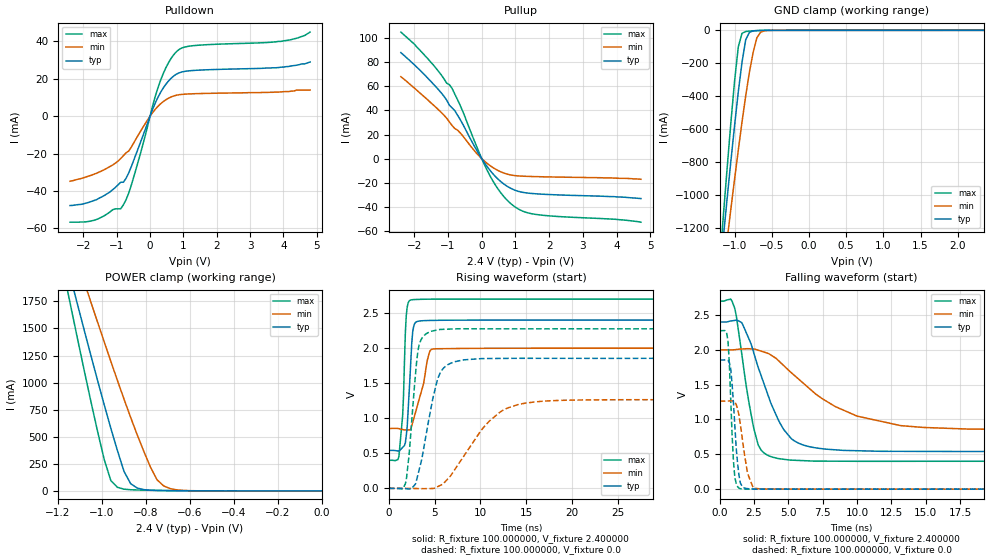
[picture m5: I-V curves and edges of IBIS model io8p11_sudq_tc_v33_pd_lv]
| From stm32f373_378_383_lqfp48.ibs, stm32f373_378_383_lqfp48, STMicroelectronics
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|   Model io8p11_sudq_tc_v33_pd_lv
[Model]  io8p11_sudq_tc_v33_pd_lv
Model_type I/O
Polarity   Non-Inverting
Enable   Active-Low
Vinl =   0.720000V
Vinh =   1.680000V
Vmeas =  1.200000V
Cref =   50.000000pF
Rref =   100.000000M
Vref =   0.0V
C_comp   1.373400pF   1.288200pF   1.481900pF
[Temperature Range]   25.000000   0.125000k   -40.000000
[Pullup Reference]   2.400000V   2.000000V   2.700000V
[Pulldown Reference]   0.0V   0.0V   0.0V
[POWER Clamp Reference]   2.400000V   2.000000V   2.700000V
[GND Clamp Reference]   0.0V   0.0V   0.0V
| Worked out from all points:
|   slope of the pulldown table from 0 to 0.36 V, typ, clamps not added: 25.7 ohm
|   slope of the pullup table from 0 to 0.36 V, typ, clamps not added: 26.8 ohm
|   GND clamp passes 1 mA (typ) near -0.67 V on its own axis
|   POWER clamp passes 1 mA (typ) near -0.60 V on its own axis
|   rising waveform, R_fixture 100.000000, V_fixture 2.400000: 20-80 % time 466ps typ, 1.22ns min, 428ps max; typ from 0.541 V to 2.4 V
|   rising waveform, R_fixture 100.000000, V_fixture 0.0: 20-80 % time 1.66ns typ, 4.33ns min, 861ps max; typ from 0 V to 1.85 V
|   falling waveform, R_fixture 100.000000, V_fixture 2.400000: 20-80 % time 2.12ns typ, 4.93ns min, 1.11ns max; typ from 2.4 V to 0.541 V
|   falling waveform, R_fixture 100.000000, V_fixture 0.0: 20-80 % time 392ps typ, 571ps min, 290ps max; typ from 1.85 V to 0 V
[Pulldown]
|Voltage   I(typ)   I(min)   I(max)
-2.4V     -47.8mA    -34.8mA    -56.7mA
-1.68V    -45.1mA    -31mA      -55.7mA
-1.12V    -39.3mA    -26.1mA    -50.03mA
-800mV    -35.33mA   -21.13mA   -47.42mA
-640mV    -30.33mA   -18.65mA   -41.16mA
-480mV    -23.12mA   -14mA      -31.94mA
240mV     10.22mA    5.339mA    15.38mA
480mV     17.22mA    8.864mA    26.1mA
800mV     22.59mA    11.27mA    34.68mA
1.36V     24.54mA    12.05mA    37.84mA
3.92V     26.2mA     13mA       40mA
4.8V      29mA       14mA       45mA
[Pullup]
|Voltage   I(typ)   I(min)   I(max)
-2.4V     88mA       68mA       105mA
-2V       77.9mA     58.6mA     95mA
-1.36V    59.6mA     42.6mA     75.1mA
-880mV    42.13mA    27.44mA    58.22mA
-560mV    28.45mA    18.75mA    39mA
-160mV    7.44mA     4.66mA     10.64mA
160mV     -6.607mA   -3.947mA   -9.704mA
480mV     -16.91mA   -9.806mA   -25.1mA
880mV     -24.89mA   -13.63mA   -37.75mA
1.2V      -27.87mA   -14.5mA    -43.37mA
1.6V      -29.13mA   -14.89mA   -46.24mA
4.72V     -33.1mA    -17.1mA    -52.7mA
[GND_clamp]
|Voltage   I(typ)   I(min)   I(max)
-2.4V     -7.358A    -6.372A    -8.78A
-1.2V     -1.489A    -1.65A     -1.416A
-1.15V    -1.254A    -1.461A    -1.124A
-1.1V     -1.024A    -1.273A    -838.2mA
-1.05V    -797.6mA   -1.088A    -563.2mA
-950mV    -374.6mA   -728.7mA   -100.8mA
-900mV    -194.3mA   -558mA     -18.03mA
-850mV    -56.96mA   -397.5mA   -7.097mA
-750mV    -3.597mA   -133.8mA   -2.788mA
-700mV    -1.53mA    -44.71mA   -1.533mA
-600mV    -249.2uA   -2.951mA   -225.1uA
2.35V     60.02uA    46.69uA    67.1uA
[POWER_clamp]
|Voltage   I(typ)   I(min)   I(max)
-2.4V     9.979A     9.967A     9.901A
-1.17V    2.182A     2.481A     1.978A
-1.14V    1.945A     2.294A     1.683A
-1.11V    1.71A      2.108A     1.391A
-1.08V    1.476A     1.923A     1.102A
-1.05V    1.245A     1.739A     819.9mA
-960mV    578.2mA    1.196A     96.06mA
-900mV    179.5mA    846.7mA    16.04mA
-870mV    67.18mA    678.8mA    10.82mA
-780mV    6.749mA    219.9mA    5.853mA
-720mV    3.355mA    46.34mA    3.808mA
0V        0A         0A         0A
[Ramp]
| variable   typ   min   max
dV/dt_r  1.11234/1.66297n   0.75852/4.32387n   1.36500/0.85538n
dV/dt_f  1.11470/2.11669n   0.68716/4.92133n   1.37915/1.10562n
R_load = 100.000000
[Rising Waveform]
R_fixture= 100.000000
V_fixture= 2.400000
V_fixture_min= 2.000000
V_fixture_max= 2.700000
|time   V(typ)   V(min)   V(max)
0s        541.2mV    853.5mV    400.3mV
1.101ns   531.1mV    851.2mV    460mV
1.502ns   583.8mV    838.7mV    1.03V
1.902ns   754.3mV    833.4mV    2.468V
2.402ns   1.828V     847.5mV    2.686V
2.603ns   2.23V      940.9mV    2.69V
2.803ns   2.345V     1.034V     2.692V
4.404ns   2.394V     1.929V     2.697V
4.805ns   2.395V     1.987V     2.698V
49.85ns   2.399V     1.999V     2.699V
[Rising Waveform]
R_fixture= 100.000000
V_fixture= 0.0
V_fixture_min= 0.0
V_fixture_max= 0.0
|time   V(typ)   V(min)   V(max)
0s        765pV      13.32nV    588.1pV
1.802ns   -3.284mV   47.69uV    66.55mV
2.202ns   -8.589mV   -93.13uV   472.5mV
3.203ns   210.1mV    -2.639mV   1.983V
4.605ns   1.147V     -2.139mV   2.24V
5.405ns   1.585V     29.24mV    2.261V
6.507ns   1.768V     145.4mV    2.27V
10.91ns   1.851V     951.5mV    2.275V
14.31ns   1.855V     1.201V     2.275V
49.85ns   1.854V     1.264V     2.275V
[Falling Waveform]
R_fixture= 100.000000
V_fixture= 2.400000
V_fixture_min= 2.000000
V_fixture_max= 2.700000
|time   V(typ)   V(min)   V(max)
0s        2.399V     1.999V     2.699V
1.101ns   2.422V     2.002V     2.592V
1.702ns   2.351V     2.012V     1.804V
2.202ns   2.123V     2.015V     1.163V
2.803ns   1.748V     1.994V     635mV
4.204ns   1.022V     1.859V     441.7mV
6.306ns   621mV      1.483V     407.5mV
9.91ns    552.1mV    1.056V     400.1mV
13.21ns   542.8mV    911.2mV    400.1mV
49.85ns   541.2mV    853.5mV    400.3mV
[Falling Waveform]
R_fixture= 100.000000
V_fixture= 0.0
V_fixture_min= 0.0
V_fixture_max= 0.0
|time   V(typ)   V(min)   V(max)
0s        1.854V     1.264V     2.275V
600.6ps   1.85V      1.265V     2.134V
800.8ps   1.732V     1.268V     1.297V
1.001ns   1.241V     1.263V     406.4mV
1.101ns   911.7mV    1.249V     167.9mV
1.301ns   373.8mV    1.153V     36.34mV
1.502ns   92.48mV    931.7mV    6.696mV
2.002ns   8.008mV    259.7mV    1.537mV
2.803ns   1.732mV    7.079mV    778.1uV
49.85ns   765pV      13.32nV    588.1pV
